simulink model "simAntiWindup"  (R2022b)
settings: Solver=ode15s  StartTime=0.0  StopTime=4*500-1  RelTol=1e-6  EnableMultiTasking=on
undefined symbols (not defined in the file or in its folder): float
libraries: simulink_need_slupdate x2, simulink x1

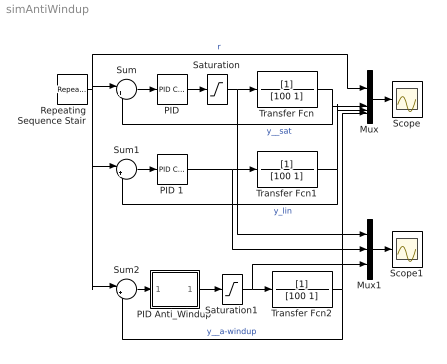
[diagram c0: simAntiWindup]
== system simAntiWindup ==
  Mux : Mux
  Mux1 : Mux  Inputs=3
  PID : simulink_need_slupdate/PID Controller  P=10  I=.5  D=10
  PID Anti_Windup : Subsystem
  PID 1 : simulink_need_slupdate/PID Controller  P=10  I=.5  D=10
  Repeating Sequence Stair : simulink/Sources/Repeating Sequence Stair  OutValues=10*[1 2 3 4 5 6].'  tsamp=500  OutMin=[]  OutMax=[]  OutDataTypeStr=float('double')  OutputDataTypeScalingMode=Specify via dialog  OutDataType=float('double')  ConRadixGroup=Best Precision: Vector-wise  OutScaling=2^-12
  Saturation : Saturate  UpperLimit=50  LowerLimit=0
  Saturation1 : Saturate  UpperLimit=50  LowerLimit=0
  Scope : Scope
  Scope1 : Scope
  Sum : Sum  Inputs=|+-
  Sum1 : Sum  Inputs=|+-
  Sum2 : Sum  Inputs=|+-
  Transfer Fcn : TransferFcn  Denominator=[100 1]
  Transfer Fcn1 : TransferFcn  Denominator=[100 1]
  Transfer Fcn2 : TransferFcn  Denominator=[100 1]
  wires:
  Repeating Sequence Stair/1 -> Sum/1, Sum1/1, Sum2/1, Mux/1  "r"
  Transfer Fcn/1 -> Sum/2, Mux/2  "y__sat"
  PID/1 -> Saturation/1
  Sum/1 -> PID/1
  Saturation/1 -> Transfer Fcn/1, Mux1/1
  Mux/1 -> Scope/1
  Transfer Fcn1/1 -> Sum1/2, Mux/3  "y_lin"
  PID 1/1 -> Transfer Fcn1/1, Mux1/2
  Sum1/1 -> PID 1/1
  Transfer Fcn2/1 -> Sum2/2, Mux/4  "y__a-windup"
  PID Anti_Windup/1(Out1) -> Saturation1/1
  Sum2/1 -> PID Anti_Windup/1(In1)
  Saturation1/1 -> Transfer Fcn2/1, Mux1/3
  Mux1/1 -> Scope1/1

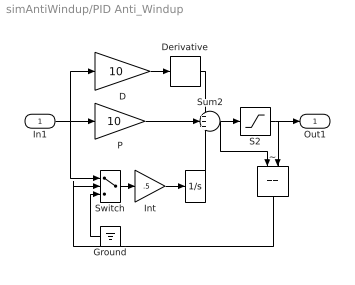
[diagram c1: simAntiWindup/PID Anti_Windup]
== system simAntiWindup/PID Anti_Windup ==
  In1 : Inport
  D : Gain  Gain=10
  Derivative : Derivative
  Ground : Ground
  I : Integrator
  Int : Gain  Gain=.5
  P : Gain  Gain=10
  S2 : Saturate  UpperLimit=50  LowerLimit=0
  Sum2 : Sum  Inputs=+++
  Switch : Switch
  ~ : RelationalOperator  Operator===  OutDataTypeStr=boolean
  Out1 : Outport
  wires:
  S2/1 -> ~/2, Out1/1
  In1/1 -> Switch/1, D/1, P/1
  D/1 -> Derivative/1
  Derivative/1 -> Sum2/1
  P/1 -> Sum2/2
  Switch/1 -> Int/1
  Ground/1 -> Switch/3
  I/1 -> Sum2/3
  Sum2/1 -> S2/1, ~/1
  ~/1 -> Switch/2
  Int/1 -> I/1
